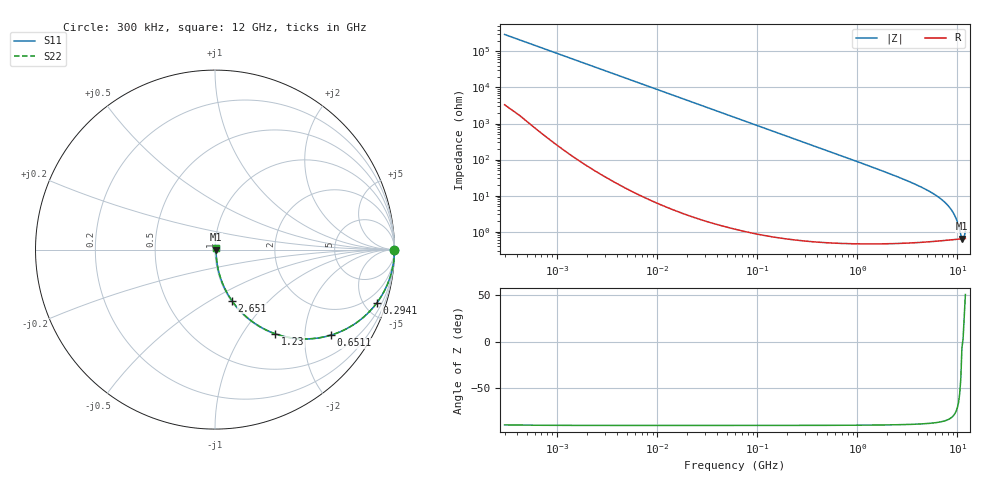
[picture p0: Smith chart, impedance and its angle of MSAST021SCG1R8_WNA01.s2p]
! MSAST021SCG1R8_WNA01  S-PARAMETER MODEL  ( General Type )
! Model Generated by TAIYO YUDEN Corporation (http://www.ty-top.com)
! Version 2.0
! TAIYO YUDEN Control No. 181101
! Copyright(c) 2015 TAIYO YUDEN CO.,LTD. All Rights Reserved.
! Product Description (link to TY-COMPAS)
! https://ds.yuden.co.jp/TYCOMPAS/or/detail?pn=MSAST021SCG1R8BWNA01&u=M
! Products Name : Multilayer Ceramic Capacitors
! Characteristics :
!  Capacitance : 1.8 pF , Rated Voltage : 25V , TCC : CG / C0G
!  Case Size : 0.25 x 0.125 / 0.0098 x 0.0049 [mm/inch] , Thickness : 0.125 / 0.0049 [mm/inch]
!  (Conditions: Temperature = 25 degC , DC Bias Current/Voltage = 0A / 0V)
! External Node Assignments :
!  1  o---| |---o  2
! GND o---------o GND
! Frequency Range : 0.3MHz  -  12000MHz  [ 401 STEP ]
# MHz S RI R 50
! Freq[MHz].  S11 Real  S11 Imag  S21 Real  S21 Imag  S12 Real  S12 Imag  S22 Real  S22 Imag
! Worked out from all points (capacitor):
!   401 points, 300 kHz to 12 GHz, reference 50 ohm
!   read as one part in series: C = 1.8 pF near 316.3 kHz
!   lowest |Z| = 639 mohm at 11.08 GHz (marker M1)
!   series resonance near 11.28 GHz, so ESL is about 110 pH
!   S11 on the Smith chart (normalised r, x): 300 kHz: open; 294.1 MHz: 1.01, -6.01; 651.1 MHz: 1.01, -2.71; 1.23 GHz: 1.01, -1.42; 2.651 GHz: 1.01, -0.63; 12 GHz: 1.01, +0.02
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0.3  1 -0.000339  3.92e-06 0.000339  3.92e-06 0.000339  1 -0.000339
1.769972  1 -0.002  7.32e-06 0.002  7.32e-06 0.002  1 -0.002
10.44266  0.9999 -0.0118  0.000148 0.0118  0.000148 0.0118  0.9999 -0.0118
60  0.9954 -0.0675  0.00464 0.0675  0.00464 0.0675  0.9954 -0.0675
140.0606  0.9753 -0.1545  0.0247 0.1545  0.0247 0.1545  0.9753 -0.1545
294.0765  0.8998 -0.2993  0.1002 0.2993  0.1002 0.2993  0.8998 -0.2993
353.9943  0.8611 -0.3448  0.1389 0.3448  0.1389 0.3448  0.8611 -0.3448
651.0506  0.6464 -0.4763  0.3536 0.4763  0.3536 0.4763  0.6464 -0.4763
894.6982  0.4909 -0.4976  0.5091 0.4976  0.5091 0.4976  0.4909 -0.4976
1229.528  0.3364 -0.4693  0.6636 0.4693  0.6636 0.4693  0.3364 -0.4693
2088.533  0.1459 -0.3473  0.8541 0.3473  0.8541 0.3473  0.1459 -0.3473
2650.866  0.0936 -0.2839  0.9064 0.2839  0.9064 0.2839  0.0936 -0.2839
5006.236  0.0244 -0.1369  0.9756 0.1369  0.9756 0.1369  0.0244 -0.1369
6188.031  0.015 -0.0969  0.985 0.0969  0.985 0.0969  0.015 -0.0969
7448.838  0.00991 -0.0648  0.9901 0.0648  0.9901 0.0648  0.00991 -0.0648
8281.503  0.00808 -0.0473  0.9919 0.0473  0.9919 0.0473  0.00808 -0.0473
9207.246  0.00691 -0.0302  0.9931 0.0302  0.9931 0.0302  0.00691 -0.0302
9708.23  0.00656 -0.0218  0.9934 0.0218  0.9934 0.0218  0.00656 -0.0218
10793.46  0.00628 -0.00525  0.9937 0.00525  0.9937 0.00525  0.00628 -0.00525
11083.22  0.0063 -0.000727  0.9937 0.000727  0.9937 0.000727  0.0063 -0.000727
11380.75  0.00635 0.000365  0.9937 -0.000365  0.9937 -0.000365  0.00635 0.000365
12000  0.0065 0.00784  0.9935 -0.00784  0.9935 -0.00784  0.0065 0.00784
